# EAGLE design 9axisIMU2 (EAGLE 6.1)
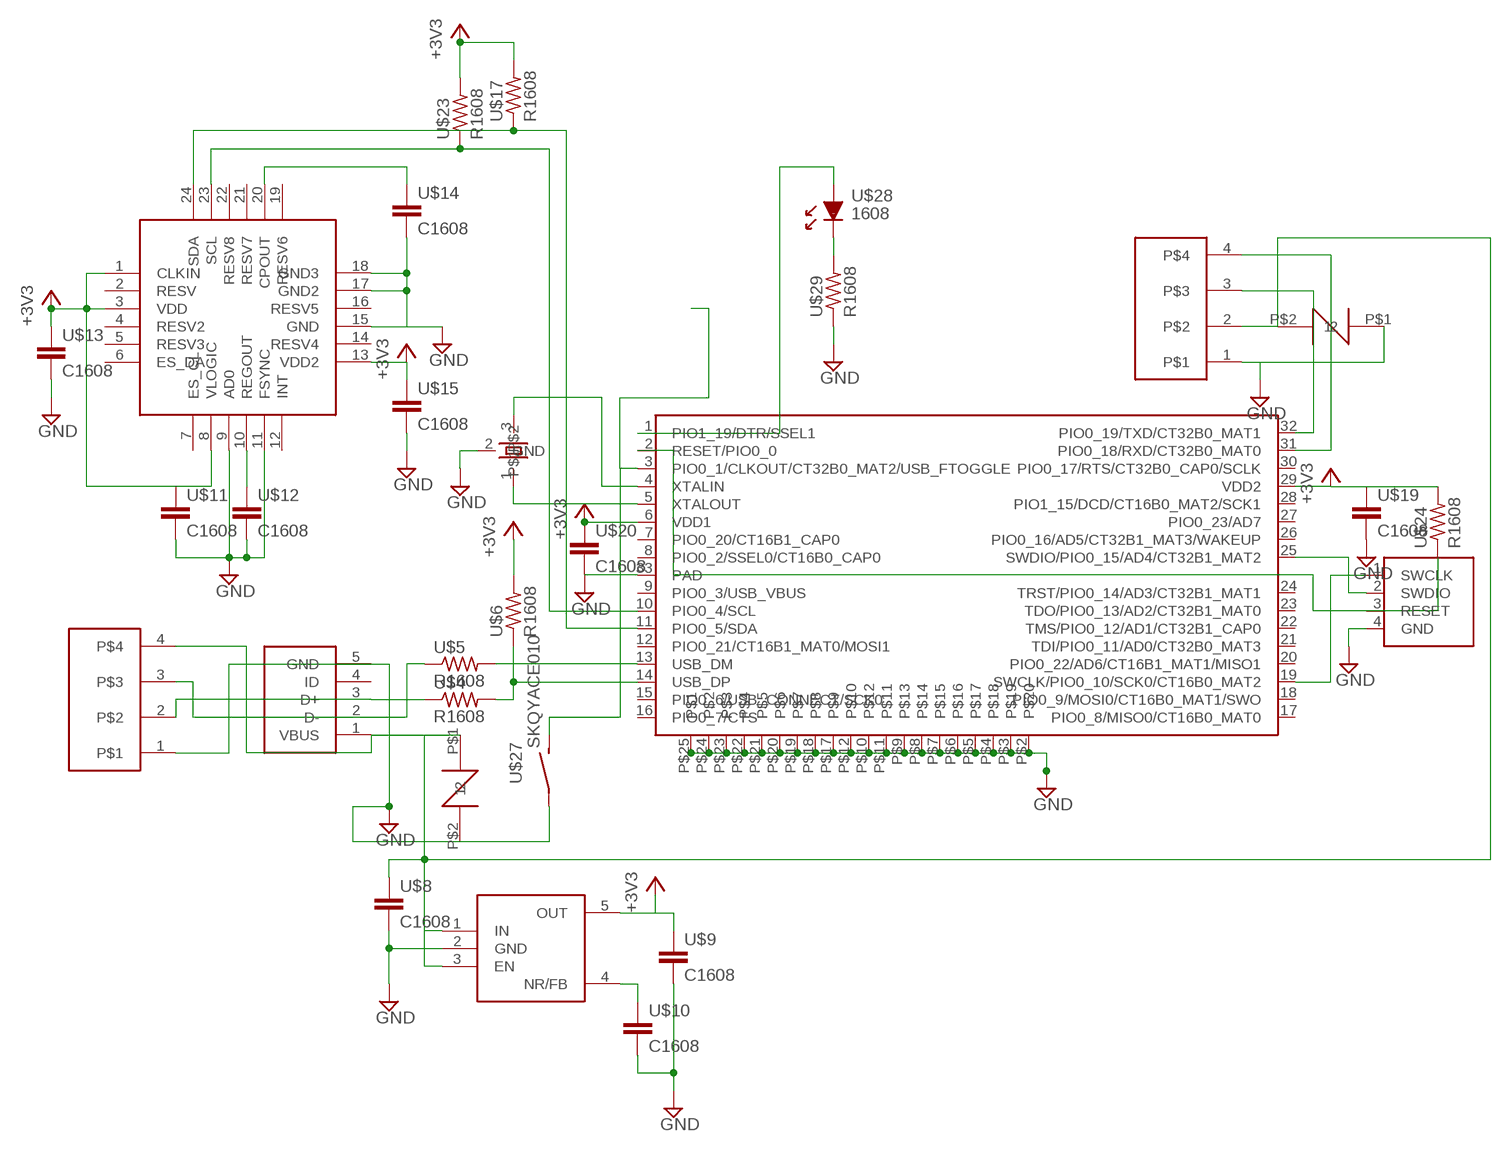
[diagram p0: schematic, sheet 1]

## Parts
U$1  LPC1315  [LPC1315]
U$2  MICROUSB  [MICROUSB]
U$3  MPU9150  [MPU9150]
U$4  R1608  [R1608]
U$5  R1608  [R1608]
U$6  R1608  [R1608]
U$7  TPS71733  [TPS71733]
U$8  C1608  [C1608]
U$9  C1608  [C1608]
U$10  C1608  [C1608]
U$11  C1608  [C1608]
U$12  C1608  [C1608]
U$13  C1608  [C1608]
U$14  C1608  [C1608]
U$15  C1608  [C1608]
U$16  DEBUG  [CONNRCTOR2]
U$17  R1608  [R1608]
U$18  2.54PIN4  [2.54PIN4]
U$19  C1608  [C1608]
U$20  C1608  [C1608]
U$21  2.54PIN4  [2.54PIN4]
U$22  CSTCE_G  [CSTCE_G]
U$23  R1608  [R1608]
U$24  R1608  [R1608]
U$25  VARISTOR  [1608]
U$26  VARISTOR  [1608]
U$27  SKQYACE010  [SKQYACE010]
U$28  1608  [1608]
U$29  R1608  [R1608]

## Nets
+3V3: U$1.6(VDD1) U$1.29(VDD2) U$3.1(CLKIN) U$3.3(VDD) U$3.8(VLOGIC) U$3.13(VDD2) U$6.P$2 U$7.5(OUT) U$9.P$1 U$11.P$1 U$13.P$1 U$15.P$1 U$17.P$2 U$19.P$1 U$20.P$1 U$23.P$2 U$24.P$2
GND: U$1.33(PAD) U$1.P$2 U$1.P$3 U$1.P$4 U$1.P$5 U$1.P$6 U$1.P$7 U$1.P$8 U$1.P$9 U$1.P$10 U$1.P$11 U$1.P$12 U$1.P$17 U$1.P$18 U$1.P$19 U$1.P$20 U$1.P$21 U$1.P$22 U$1.P$23 U$1.P$24 U$1.P$25 U$2.5(GND) U$3.9(AD0) U$3.11(FSYNC) U$3.15(GND) U$3.17(GND2) U$3.18(GND3) U$7.2(GND) U$8.P$2 U$9.P$2 U$10.P$2 U$11.P$2 U$12.P$2 U$13.P$2 U$14.P$2 U$15.P$2 U$16.4(GND) U$18.1 U$19.P$2 U$20.P$2 U$21.1 U$22.2(GND) U$25.P$2 U$26.P$1 U$27.P$1(P) U$29.P$1
N$2: U$1.13(USB_DM) U$5.P$2
N$3: U$2.2(D-) U$5.P$1 U$21.3
N$4: U$2.3(D+) U$4.P$1 U$21.2
N$5: U$1.14(USB_DP) U$4.P$2 U$6.P$1
N$6: U$2.1(VBUS) U$7.1(IN) U$7.3(EN) U$8.P$1 U$18.2 U$21.4 U$25.P$1 U$26.P$2
N$7: U$7.4(NR/FB) U$10.P$1
N$8: U$3.10(REGOUT) U$12.P$1
N$9: U$3.20(CPOUT) U$14.P$1
N$11: U$1.10(PIO0_4/SCL) U$3.23(SCL) U$23.P$1
N$12: U$1.11(PIO0_5/SDA) U$3.24(SDA) U$17.P$1
N$13: U$1.19(SWCLK/PIO0_10/SCK0/CT16B0_MAT2) U$16.1(SWCLK)
N$14: U$1.25(SWDIO/PIO0_15/AD4/CT32B1_MAT2) U$16.2(SWDIO)
N$15: U$1.2(RESET/PIO0_0) U$16.3(RESET) U$24.P$1
N$16: U$1.3(PIO0_1/CLKOUT/CT32B0_MAT2/USB_FTOGGLE) U$27.P$2(S)
N$17: U$1.32(PIO0_19/TXD/CT32B0_MAT1) U$18.3
N$18: U$1.31(PIO0_18/RXD/CT32B0_MAT0) U$18.4
N$19: U$1.4(XTALIN) U$22.3
N$20: U$1.5(XTALOUT) U$22.1
N$23: U$1.1(PIO1_19/DTR/SSEL1) U$28.1(A)
N$24: U$28.2(K) U$29.P$2
Unconnected: U$1.7(PIO0_20/CT16B1_CAP0) U$1.8(PIO0_2/SSEL0/CT16B0_CAP0) U$1.9(PIO0_3/USB_VBUS) U$1.12(PIO0_21/CT16B1_MAT0/MOSI1) U$1.15(PIO0_6/USB_CONNECT/SCK0) U$1.16(PIO0_7/CTS) U$1.17(PIO0_8/MISO0/CT16B0_MAT0) U$1.18(PIO0_9/MOSI0/CT16B0_MAT1/SWO) U$1.20(PIO0_22/AD6/CT16B1_MAT1/MISO1) U$1.21(TDI/PIO0_11/AD0/CT32B0_MAT3) U$1.22(TMS/PIO0_12/AD1/CT32B1_CAP0) U$1.23(TDO/PIO0_13/AD2/CT32B1_MAT0) U$1.24(TRST/PIO0_14/AD3/CT32B1_MAT1) U$1.26(PIO0_16/AD5/CT32B1_MAT3/WAKEUP) U$1.27(PIO0_23/AD7) U$1.28(PIO1_15/DCD/CT16B0_MAT2/SCK1) U$1.30(PIO0_17/RTS/CT32B0_CAP0/SCLK) U$2.4(ID) U$3.2(RESV) U$3.4(RESV2) U$3.5(RESV3) U$3.6(ES_DA) U$3.7(ES_CL) U$3.12(INT) U$3.14(RESV4) U$3.16(RESV5) U$3.19(RESV6) U$3.21(RESV7) U$3.22(RESV8)

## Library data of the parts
U$1 = LPC1315:LPC1315
U$2 = USB:MICROUSB
U$3 = gyro:MPU9150
U$4-U$6 U$17 U$23 U$24 U$29 = resistor:R1608
U$7 = regulator:TPS71733
U$8-U$15 U$19 U$20 = capacitor:C1608
U$16 = connector:DEBUG
U$18 U$21 = connector:2.54PIN4
U$22 = xtal:CSTCE_G
U$25 U$26 = fuse:VARISTOR
U$27 = sw:SKQYACE010
U$28 = LED:1608

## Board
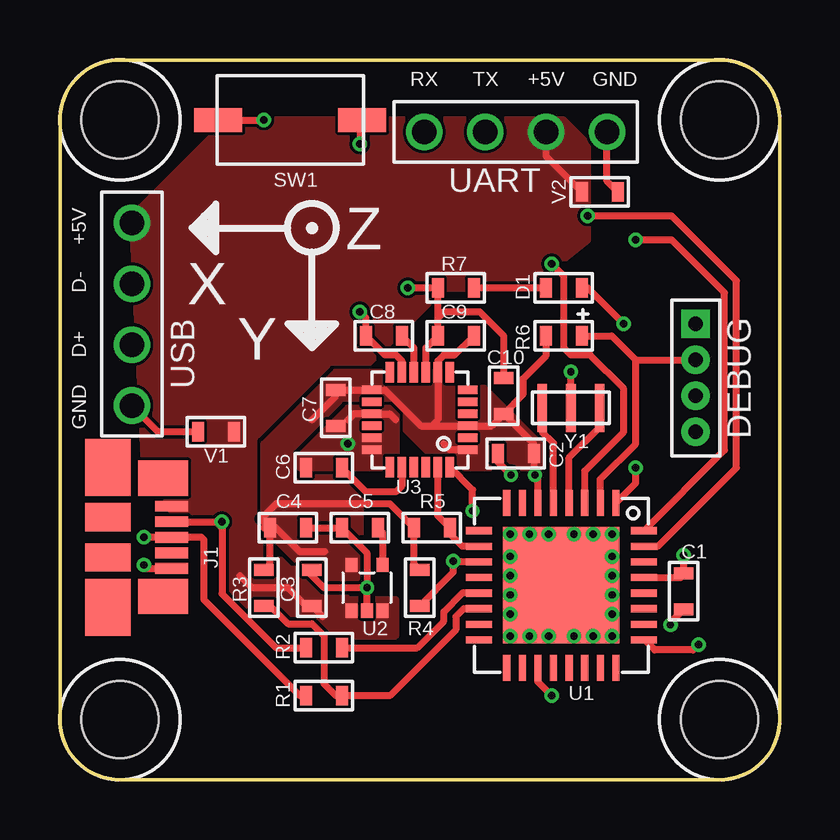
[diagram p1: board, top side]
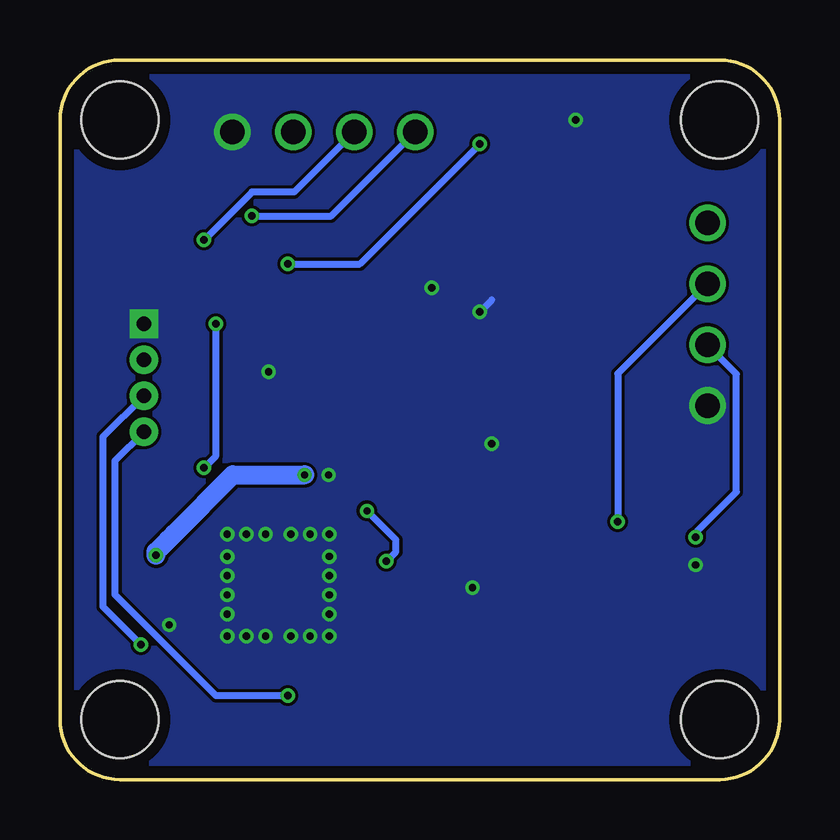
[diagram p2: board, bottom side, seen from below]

Size 30 x 30 mm. Coordinates in mm from the lower left corner, seen from the top.
Outline: 2.5,30 27.5,30 arc-90 30,27.5 30,2.5 arc-90 27.5,0 2.5,0 arc-90 0,2.5 0,27.5 arc-90 2.5,30
Copper layers (1*16): Top 0.035mm / dielectric 1.53mm / Bottom 0.035mm
Design rules: minimum track width 5mil, minimum drill 0.3mm, track to track 5mil, track to pad 0.229mm, pad to pad 5mil, via to via 5mil, smd to smd 5mil, copper to edge 0.5mm, drill to drill 0.5mm, minimum pad ring 0.15mm, minimum via ring 0.15mm, stop-mask expansion 4mil, vias tented up to drill 0.35mm, thermal gap 10mil
Holes 3.2 mm at 2.5,2.5 27.5,2.5 27.5,27.5 2.5,27.5

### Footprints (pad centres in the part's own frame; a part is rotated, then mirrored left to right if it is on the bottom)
LPC1315 = smd 1.075 x 0.3: 1 -3.438,2.275; 2 -3.438,1.625; 3 -3.438,0.975; 4 -3.438,0.325; 5 -3.438,-0.325; 6 -3.438,-0.975; 7 -3.438,-1.625; 8 -3.438,-2.275; 17 3.438,-2.275; 18 3.438,-1.625; 19 3.438,-0.975; 20 3.438,-0.325; 21 3.438,0.325; 22 3.438,0.975; 23 3.438,1.625; 24 3.438,2.275 | smd 0.3 x 1.075: 9 -2.275,-3.438; 10 -1.625,-3.438; 11 -0.975,-3.438; 12 -0.325,-3.438; 13 0.325,-3.438; 14 0.975,-3.438; 15 1.625,-3.438; 16 2.275,-3.438; 25 2.275,3.438; 26 1.625,3.438; 27 0.975,3.438; 28 0.325,3.438; 29 -0.325,3.438; 30 -0.975,3.438; 31 -1.625,3.438; 32 -2.275,3.438 | smd 4.85 x 4.85: 33 0,0 | drill 0.3 pad 0.6: P$2 -1.2,-2.125; P$3 1.2,-2.125; P$4 -0.4,-2.125; P$5 0.4,-2.125; P$6 2.125,-2.125; P$7 -2.125,-2.125; P$8 2.125,0.525; P$9 2.125,-0.525; P$10 2.125,-1.325; P$11 2.125,1.325; P$12 2.125,2.125; P$17 -2.125,1.325; P$18 -2.125,2.125; P$19 -2.125,-1.325; P$20 -2.125,-0.525; P$21 -2.125,0.525; P$22 0.4,2.125; P$23 -0.4,2.125; P$24 -1.2,2.125; P$25 1.2,2.125
MICROUSB = smd 0.45 x 1.38: 1 1.3,-2.66; 2 0.65,-2.66; 3 0,-2.66; 4 -0.65,-2.66; 5 -1.3,-2.66 | smd 2.375 x 1.9: P$1 2.913,0; P$2 -2.913,0 | smd 1.175 x 1.9: P$3 0.838,0; P$4 -0.838,0 | smd 1.475 x 2.1: P$5 2.462,-2.3; P$6 -2.462,-2.3
MPU9150 = smd 0.8 x 0.35: 1 -2,1.25; 2 -2,0.75; 3 -2,0.25; 4 -2,-0.25; 5 -2,-0.75; 6 -2,-1.25; 13 2,-1.25; 14 2,-0.75; 15 2,-0.25; 16 2,0.25; 17 2,0.75; 18 2,1.25 | smd 0.35 x 0.85: 7 -1.25,-1.975; 8 -0.75,-1.975; 9 -0.25,-1.975; 10 0.25,-1.975; 11 0.75,-1.975; 12 1.25,-1.975; 19 1.25,1.975; 20 0.75,1.975; 21 0.25,1.975; 22 -0.25,1.975; 23 -0.75,1.975; 24 -1.25,1.975
R1608 = smd 0.5 x 0.8: P$1 0.75,0; P$2 -0.75,0
TPS71733 = smd 0.5 x 0.6: 1 -0.65,-0.95; 2 0,-0.95; 3 0.65,-0.95; 4 0.65,0.95; 5 -0.65,0.95
C1608 = smd 0.5 x 0.8: P$1 0.75,0; P$2 -0.75,0
CONNRCTOR2 = drill 0.6 pad 1.2: 1 3,0; 2 1.5,0; 3 0,0 | drill 0.6 pad 1.2 square: 4 -1.5,0
2.54PIN4 = drill 1.02: 1 -3.81,0; 2 -1.27,0; 3 1.27,0; 4 3.81,0
CSTCE_G = smd 0.4 x 2: 1 -1.2,0; 2 0,0; 3 1.2,0
1608 = smd 0.5 x 0.8: P$1 0.75,0; P$2 -0.75,0
SKQYACE010 = smd 2 x 1: P$1 -3,0; P$2 3,0
1608' = smd 0.5 x 0.8: 1 -0.75,0; 2 0.75,0

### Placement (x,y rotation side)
U$1  20.9,8.1 270 top
U$2  2,10.1 90 top
U$3  15,15 180 top
U$4  11,3.5 180 top
U$5  11,5.5 180 top
U$6  8.5,8 270 top
U$7  12.8,8 0 top
U$8  10.5,8 270 top
U$9  9.5,10.5 180 top
U$10  12.5,10.5 0 top
U$11  16.5,18.5 0 top
U$12  13.5,18.5 0 top
U$13  11.5,15.5 90 top
U$14  11,13 0 top
U$15  26,7.85 90 top
U$16  26.5,17.5 270 top
U$17  15,8 270 top
U$18  19,27 180 top
U$19  19,13.6 0 top
U$20  18.5,16 270 top
U$21  3,19.4 90 top
U$22  21.3,15.5 0 top
U$23  15.5,10.5 0 top
U$24  21,18.5 0 top
U$25  6.5,14.5 0 top
U$26  22.5,24.5 0 top
U$27  9.6,27.5 0 top
U$28  1608  [1608']  21,20.5 180 top
U$29  16.5,20.5 180 top

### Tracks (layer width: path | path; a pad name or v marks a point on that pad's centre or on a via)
+3V3  (via drill 0.3 pad 0.6)
  Top 0.3: 8.5,10.5 U$9.P$1 | U$1.6 19.93,12.57 v19.8,12.7 19.75,12.75 U$19.P$1 19.75,14 U$20.P$1 | U$9.P$1 9,10.5 10,9.5 11.05,9.5 | U$20.P$1 18,14.75 U$3.3 15.5,14.75 | 8.75,10.75 U$9.P$1 | U$13.P$1 U$3.13 13.55,16.25 15.05,14.75 15.5,14.75 | 11.25,16.25 U$13.P$1 | U$9.P$1 8.38,10.88 9,11.5 13.75,11.5 U$23.P$2 14.75,9 U$17.P$2 | v26,9.35 U$15.P$1 25.88,8.43 U$1.29 | 10.5,15 11.5,16 U$13.P$1 | U$24.P$2 20.25,17.65 19.3,16.7 19.3,16.05 U$20.P$1 | U$11.P$1 16.45,17.7 16,17.7 15.75,17.45 U$3.8 15.75,15 15.5,14.75 | U$6.P$2 8.75,9 U$9.P$1 | U$3.1 16.25,13.75 16,14
  Bottom 0.8: v19.8,12.7 22.8,12.7 25.25,10.25 25.5,10 26,9.5 v26,9.35
  pour Top (rank 2, no thermals): 12.5,8.3 10.7,8.3 8.5,10.5 8.5,14 11.5,17 17,17 20,14 20,13 16,13 13.5,15.5 12,15.5 10.5,14 12.5,12
GND  (via drill 0.3, 0.3 pad 0.6)
  Top 0.3: U$8.P$2 10.25,8.75 11,8 v12.8,8 | v12.8,8 12.8,9.45 U$10.P$2 U$9.P$2 10.25,10.75 | 10.25,12.75 U$14.P$2 | U$22.2 v21.3,17 | 18.25,13.65 U$19.P$2 18.25,13.25 v18.8,12.7 | v12.8,8 12.9,8 | U$3.11 14.25,17.45 14,17.7 13.55,17.7 U$12.P$2 12.75,19.25 v12.5,19.5 | U$3.9 15.25,18 U$11.P$2 15.75,19.25 | U$20.P$2 18.5,18.5 17.5,19.5 16,19.5 15.75,19.25 | U$1.P$9 U$1.P$10 U$1.P$6 U$1.P$3 U$1.P$5 | U$1.P$5 U$1.P$4 U$1.P$2 U$1.P$7 U$1.P$19 U$1.P$20 U$1.P$21 U$1.P$17 U$1.P$18 U$1.P$24 U$1.P$23 U$1.P$22 U$1.P$25 U$1.P$12 U$1.P$11 U$1.P$8 | U$1.33 19.27,8 U$1.P$5 | U$26.P$1 22.81,24.94 U$18.1 | U$27.P$1 v8.5,27.5 | v3.5,8.95 3.65,8.8 U$2.5 | U$25.P$2 4.09,14.5 U$21.1 | U$15.P$2 25.45,6.55 v25.45,6.45 | U$7.2 v12.8,8 | 14,15 13.75,15.25 U$3.15 12.25,15.25 12,15 | v14.5,20.5 U$29.P$1 15.75,19.25
  Bottom 0.3: v12.5,19.5 12,20
  other vias: 12,14
  pour Bottom (no thermals): 0,30 30,30 30,0 0,0
  pour Top (no thermals): 14,13 10,13 10,13.5 12,15.5 14,15.5
N$2
  Top 0.3: U$1.13 16.77,7.78 16,7 16,6.6 14.9,5.5 U$5.P$2
N$3  (via drill 0.3)
  Top 0.3: U$5.P$1 9,5.5 6.75,7.75 v6.75,10.75 6.75,10.5 6.5,10.75 U$2.2
  Bottom 0.3: U$21.3 6.75,16.92 v6.75,10.75
N$4  (via drill 0.3 pad 0.6)
  Top 0.3: v3.5,10.1 U$2.3 5.9,10.1 6,10 6,7.5 10,3.5 U$4.P$1
  Bottom 0.3: v3.5,10.1 3.5,10.3 1.8,12 1.8,16.9 3,18.1 U$21.2
N$5
  Top 0.3: U$6.P$1 8.75,7.25 9.5,6.5 10.5,6.5 11,6 11,4 11.5,3.5 U$4.P$2 13.75,3.5 16.5,6.25 16.5,6.8 16.82,7.12 U$1.14
N$6
  Top 0.3: U$18.2 20.27,25.98 U$26.P$2 | 10.95,6.8 U$8.P$1 10.25,7.25 9.5,8 8,8 7.5,8.5
  pour Top (rank 3, no thermals): 22,26.5 21,27.5 7,27.5 3,23.5 3.5,13 8,6 14,6 14,7.5 12,7.5 9.5,12 9.5,14 16,20.5 19.5,20.5 22,22.5
N$7
  Top 0.3: U$10.P$1 13.45,10.3 U$7.4
N$8
  Top 0.3: U$3.10 14.75,18 U$12.P$1
N$9
  Top 0.3: U$3.20 14.25,12.25 14,12 12.75,12 U$14.P$1
N$11
  Top 0.3: U$1.10 16.77,9.72 16.25,10.25 U$23.P$1 15.75,11 U$3.23
N$12  (via drill 0.3 pad 0.6)
  Top 0.3: U$1.11 16.52,9.07 v16.4,9.1 16.4,8.65 U$17.P$1 | v17.2,11.2 17.2,12.07 U$3.24
  Bottom 0.3: v16.4,9.1 16,9.5 16,10 v17.2,11.2
N$13  (via drill 0.3 pad 0.6)
  Top 0.3: U$1.19 19.93,4.07 v20.5,3.5
  Bottom 0.3: v20.5,3.5 23.5,3.5 27.7,7.7 27.7,13.3 U$16.1
N$14  (via drill 0.3 pad 0.6)
  Top 0.3: v26.62,5.62 26.4,5.4 24.8,5.4 24.38,5.82 U$1.25
  Bottom 0.3: U$16.2 28.2,14.3 28.2,7.2 v26.62,5.62
N$15
  Top 0.3: U$1.2 22.52,12.53 24,14 24,17.5 | 24,17.5 U$16.3 | U$24.P$1 23,18.5 24,17.5
N$16  (via drill 0.3)
  Top 0.3: U$1.3 21.88,12.88 23.5,14.5 23.5,16.3 22.1,17.7 21.3,17.7 21,18 21,21 v20.5,21.5 | U$27.P$2 12.5,27.4 v12.5,26.5
  Bottom 0.3: v12.5,26.5 17.5,21.5 v20.5,21.5
N$17  (via drill 0.3)
  Top 0.3: U$1.32 27.7,13.74 27.7,20.3 25.5,22.5 v24,22.5
  Bottom 0.3: U$18.3 20.23,24.5 22,24.5 v24,22.5
N$18  (via drill 0.3)
  Top 0.3: U$1.31 24.93,9.72 28.2,13 28.2,20.8 25.5,23.5 v22,23.5
  Bottom 0.3: v22,23.5 18.69,23.5 U$18.4
N$19
  Top 0.3: U$1.4 21.23,13.43 22.5,14.7 U$22.3
N$20
  Top 0.3: U$1.5 20.57,14.03 20.1,14.5 U$22.1
N$23  (via drill 0.3 pad 0.6)
  Top 0.3: U$28.1 22,20.5 v23.5,19 | U$1.1 24,12.36 v24,13
  Bottom 0.3: v24,13 23.5,13.5 v23.5,19
N$24
  Top 0.3: U$28.2 U$29.P$2

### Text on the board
tPlace: RX | TX | +5V | GND | SW1 | UART | V2 | +5V | Z | R7 | D- | X | D1 | C8 | C9 | D+ | R6 | Y | C10 | USB | GND | C7 | Y1 | DEBUG | V1 | C6 | C2 | U3 | C4 | C5 | R5 | J1 | C1 | R3 | C3 | U2 | R4 | R2 | R1 | U1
